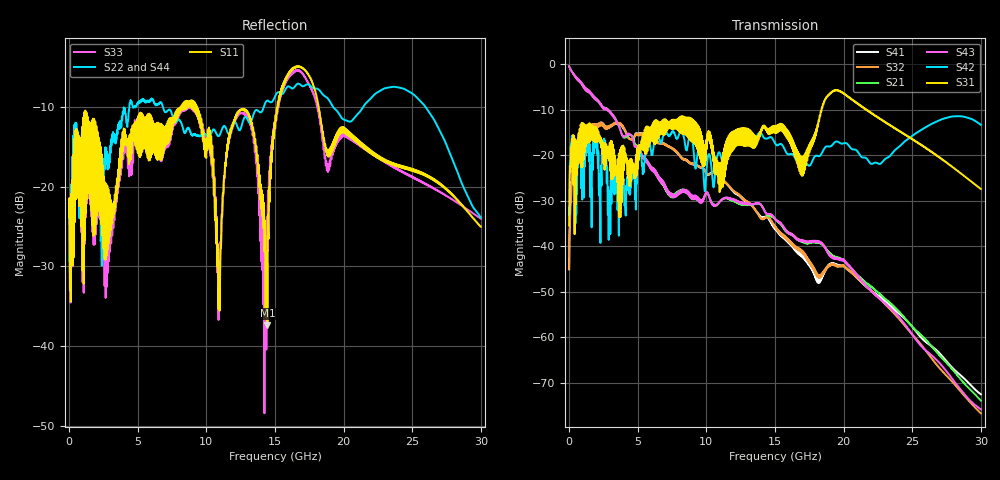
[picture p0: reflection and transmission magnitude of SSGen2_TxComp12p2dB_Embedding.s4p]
# Hz S RI R 50
! S-Parameters data
! Freq  reS11  imS11  reS12  imS12  reS13  imS13  reS14  imS14
!  reS21  imS21  reS22  imS22  reS23  imS23  reS24  imS24
!  reS31  imS31  reS32  imS32  reS33  imS33  reS34  imS34
!  reS41  imS41  reS42  imS42  reS43  imS43  reS44  imS44
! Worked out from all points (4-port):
!   1500 points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, 20 MHz to 30 GHz, reference 50 ohm
!   strongest paths, dB at 20 MHz, 7.52 GHz, 15.02 GHz, 22.52 GHz, 30 GHz:
!     S31: -35.5, -12.7, -13.5, -11.7, -27.4
!     S42: -33.2, -14.9, -17.4, -21.8, -13.3
!     S43: -0.4, -28.6, -34.1, -51.3, -75.9
!     S21: -0.4, -28.9, -34.1, -50.2, -74.0
!     S32: -45.1, -18.6, -35.7, -51.2, -76.7
!     S41: -45.1, -18.6, -36.2, -50.8, -72.6
!   lowest |S11| = -37.4 dB at 14.46 GHz (marker M1), VSWR 1.03, Z = 50.2 + j1.33 ohm
!   |S11| at or under -10 dB: start of sweep to 8.17 GHz; 9.322 GHz to 15.2 GHz (5.873 GHz wide, 47.9 % of centre); 18.19 GHz to end of sweep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
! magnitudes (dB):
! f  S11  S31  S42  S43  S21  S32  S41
! 20 MHz  -23.8  -35.5  -33.2  -0.4  -0.4  -45.1  -45.1
! 2.34 GHz  -17.0  -16.2  -22.3  -8.9  -8.9  -13.5  -13.4
! 10.94 GHz  -32.8  -21.8  -19.3  -30.4  -30.4  -24.4  -24.4
! 12.8 GHz  -10.5  -16.6  -16.7  -30.6  -30.8  -29.9  -30.1
! 14.46 GHz  -37.4  -14.2  -16.3  -33.0  -33.2  -33.6  -33.7
! 16.62 GHz  -5.0  -19.1  -21.6  -38.5  -38.4  -40.2  -40.9
! 30 GHz  -25.0  -27.4  -13.3  -75.9  -74.0  -76.7  -72.6
